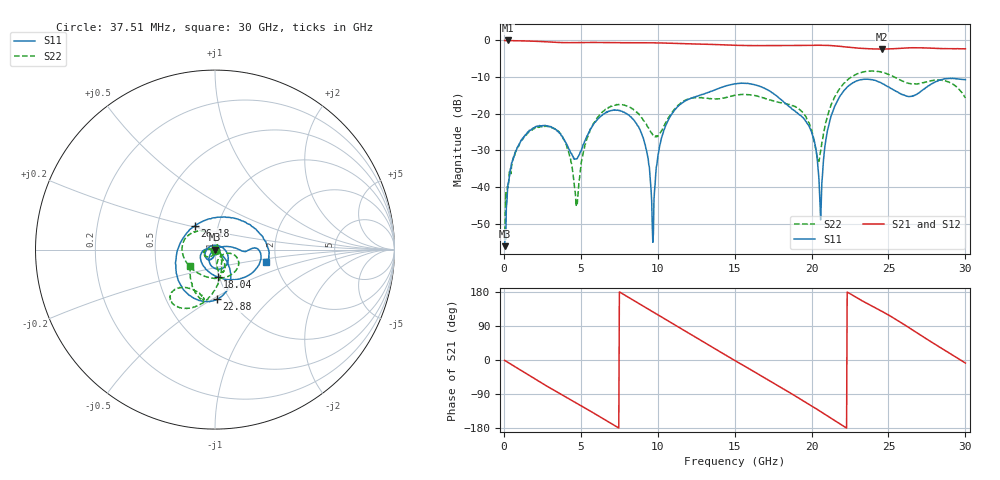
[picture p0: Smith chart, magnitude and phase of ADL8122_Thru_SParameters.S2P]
! "Analog Devices, Inc."
! Device:	ADL8122ACPZN - THRU
! Description:	"10 kHz to 10 GHz, Wideband, Low Noise Amplifier"
! Conditions:	Pin = -25 dBm
!		Operating Temperature = +25 C (at package bottom)
! Measurement used thru-cal line of SN#1.
! Frequency (GHz)	S11_Mag (dB)	S11_Phase (deg)	S21_Mag (dB)	S21_Phase (deg)	S12_Mag (dB)	S12_Phase (deg)	S22_Mag (dB)	S22_Phase (deg)
#  GHZ  S  DB  R 50
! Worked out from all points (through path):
!   800 points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, 37.51 MHz to 30 GHz, reference 50 ohm
!   highest |S21| = 0.00 dB at 262.5 MHz (marker M1); lowest = -2.3 dB at 24.56 GHz (marker M2)
!   group delay of S21, straight-line fit = 67.1 ps
!   lowest |S11| = -56.1 dB at 37.51 MHz (marker M3), VSWR 1.00, Z = 50.1 - j0.128 ohm
!   |S11| at or under -10 dB: start of sweep to end of sweep
!   |S22| runs from -54.5 to -8.3 dB; largest |S21 - S12| = 0.0047
!   S11 on the Smith chart (normalised r, x): 37.51 MHz: 1.00, -0.00; 18.04 GHz: 0.98, -0.31; 22.88 GHz: 0.88, -0.52; 26.18 GHz: 0.77, +0.21; 30 GHz: 1.77, -0.26
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0.03750899  -56.14 -54.8  -0.01 -0.9  -0.02 -1.0  -54.51 -86.1
0.2625089  -38.96 -78.4  0.01 -6.7  -0.04 -6.7  -40.16 -85.9
1.950008  -23.87 -118.0  -0.20 -48.6  -0.20 -48.6  -24.12 -142.3
3.750008  -26.03 -172.6  -0.57 -91.4  -0.58 -91.4  -26.07 -177.5
4.687507  -32.30 87.4  -0.58 -112.9  -0.58 -112.9  -45.28 -141.6
5.062508  -29.48 34.0  -0.56 -121.7  -0.56 -121.7  -32.44 -50.0
6.225007  -20.91 -34.4  -0.55 -149.7  -0.55 -149.7  -20.27 -55.9
8.137506  -20.43 -101.3  -0.61 164.4  -0.61 164.5  -18.13 -79.0
9.150006  -28.13 -134.0  -0.63 140.0  -0.63 140.1  -22.20 -81.4
9.675006  -55.09 140.1  -0.64 127.2  -0.65 127.2  -25.76 -62.3
10.05001  -30.59 27.0  -0.66 118.0  -0.67 118.0  -25.80 -36.2
11.40001  -17.63 0.6  -0.82 85.2  -0.82 85.2  -17.43 -21.7
15.0375  -11.86 -5.5  -1.31 -2.1  -1.31 -2.1  -14.99 -164.7
18.0375  -16.22 -84.4  -1.38 -73.1  -1.39 -73.1  -17.01 132.8
20.025  -25.36 179.4  -1.32 -121.8  -1.32 -121.7  -24.93 93.6
20.5875  -48.97 -102.0  -1.31 -136.1  -1.31 -136.1  -30.23 -22.3
21.3375  -19.82 -46.2  -1.42 -155.6  -1.42 -155.6  -17.01 -76.9
22.875  -11.16 -87.7  -2.05 165.7  -2.04 165.7  -9.31 -110.6
24.5625  -11.68 -143.1  -2.34 128.6  -2.34 128.5  -8.68 -132.8
25.0125  -12.68 -161.6  -2.31 118.4  -2.31 118.4  -9.28 -135.0
26.175  -15.16 130.5  -2.04 89.5  -2.05 89.5  -11.55 -126.8
30  -10.68 -13.2  -2.28 -8.0  -2.29 -8.0  -15.67 -147.3
